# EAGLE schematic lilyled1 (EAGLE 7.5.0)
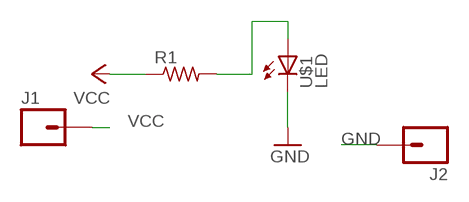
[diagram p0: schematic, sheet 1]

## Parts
J1  M01NOSILK-KIT  [1X01NS-KIT]
J2  M01NOSILK-KIT  [1X01NS-KIT]
R1  RES-US1206W  [R1206W]
U$1  LED  [LED1206]

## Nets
GND: J2.1 U$1.2(C)
N$1: R1.2 U$1.1(A)
VCC: J1.1 R1.1

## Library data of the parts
J1 J2 = SparkFun-Connectors:M01: Header 1
R1 = fab:RES-US: Resistor (US Symbol)
U$1 = fab:LED: LED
